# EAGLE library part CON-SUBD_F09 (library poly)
SUB-D
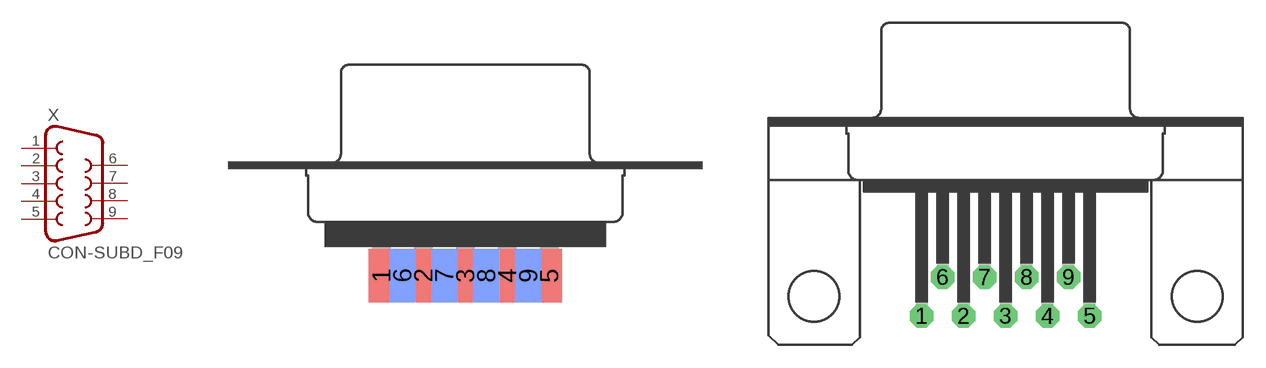
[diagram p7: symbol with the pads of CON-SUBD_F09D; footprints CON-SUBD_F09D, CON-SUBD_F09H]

Designator prefix X

## CON-SUBD_F09D (OC_FARNELL: unknown; OC_NEWARK: unknown)  [CON-SUBD_F09D]
1  1  pas
2  2  pas
3  3  pas
4  4  pas
5  5  pas
6  6  pas
7  7  pas
8  8  pas
9  9  pas

## CON-SUBD_F09H (OC_FARNELL: unknown; OC_NEWARK: unknown)  [CON-SUBD_F09H]
Pads as for CON-SUBD_F09D

## CON-SUBD_F09HP (OC_FARNELL: unknown; OC_NEWARK: unknown)  [CON-SUBD_F09HP]
Pads as for CON-SUBD_F09D

## CON-SUBD_F09V (OC_FARNELL: unknown; OC_NEWARK: unknown)  [CON-SUBD_F09V]
Pads as for CON-SUBD_F09D

## CON-SUBD_F09VB (OC_FARNELL: unknown; OC_NEWARK: unknown)  [CON-SUBD_F09VB]
Pads as for CON-SUBD_F09D

## CON-SUBD_F09VP (OC_FARNELL: unknown; OC_NEWARK: unknown)  [CON-SUBD_F09VP]
Pads as for CON-SUBD_F09D

## Footprint CON-SUBD_F09D (pad centres in mm)
SUB-D
smd 1.7 x 3.5: 1 -5.486,-6.045; 2 -2.743,-6.045; 3 0,-6.045; 4 2.743,-6.045; 5 5.486,-6.045
smd 1.7 x 3.5 bottom: 6 -4.115,-6.045; 7 -1.372,-6.045; 8 1.372,-6.045; 9 4.115,-6.045

## Footprint CON-SUBD_F09H (pad centres in mm)
SUB-D
drill 1.016 octagon: 1 -5.486,-1.27; 2 -2.743,-1.27; 3 0,-1.27; 4 2.743,-1.27; 5 5.486,-1.27; 6 -4.115,1.27; 7 -1.372,1.27; 8 1.372,1.27; 9 4.115,1.27
hole 3.302 at -12.522,0
hole 3.302 at 12.522,0

## Footprint CON-SUBD_F09HP (pad centres in mm)
SUB-D
drill 1.016 octagon: 1 -5.486,-1.27; 2 -2.743,-1.27; 3 0,-1.27; 4 2.743,-1.27; 5 5.486,-1.27; 6 -4.115,1.27; 7 -1.372,1.27; 8 1.372,1.27; 9 4.115,1.27
drill 3.302 pad 5.08: G1 -12.522,0; G2 12.522,0

## Footprint CON-SUBD_F09V (pad centres in mm)
SUB-D
drill 1.016 octagon: 1 5.486,1.422; 2 2.743,1.422; 3 0,1.422; 4 -2.743,1.422; 5 -5.486,1.422; 6 4.115,-1.422; 7 1.372,-1.422; 8 -1.372,-1.422; 9 -4.115,-1.422
hole 3.302 at -12.522,0
hole 3.302 at 12.522,0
